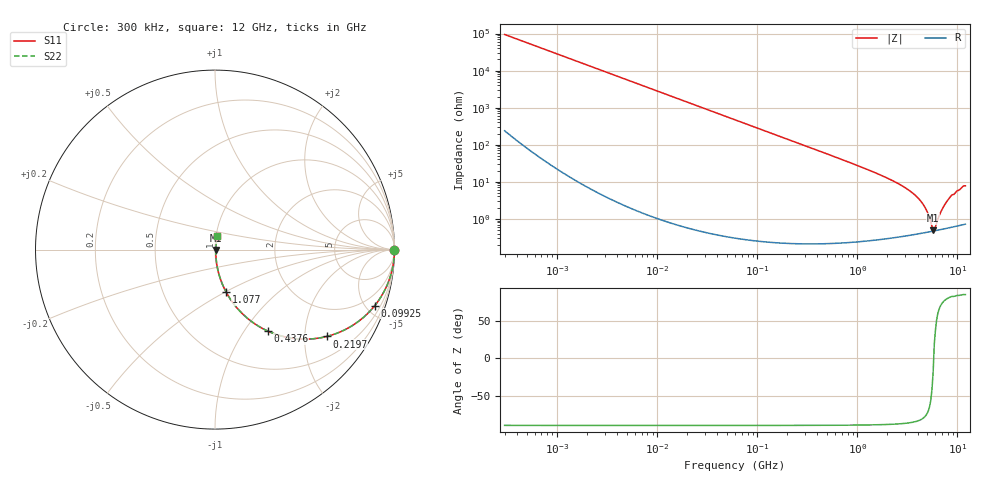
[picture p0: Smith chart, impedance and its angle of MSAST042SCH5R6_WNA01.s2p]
! MSAST042SCH5R6_WNA01  S-PARAMETER MODEL  ( General Type )
! Model Generated by TAIYO YUDEN Corporation (http://www.ty-top.com)
! Version 1.0
! TAIYO YUDEN Control No. 150820
! Copyright(c) 2015 TAIYO YUDEN CO.,LTD. All Rights Reserved.
! Product Description (link to TY-COMPAS)
! https://ds.yuden.co.jp/TYCOMPAS/or/detail?pn=MSAST042SCH5R6BWNA01&u=M
! Products Name : Multilayer Ceramic Capacitors
! Characteristics :
!  Capacitance : 5.6 pF , Rated Voltage : 25V , TCC : CH / C0H
!  Case Size : 0.4 x 0.2 / 0.016 x 0.008 [mm/inch] , Thickness : 0.2 / 0.008 [mm/inch]
!  (Conditions: Temperature = 25 degC , DC Bias Current/Voltage = 0A / 0V)
! External Node Assignments :
!  1  o---| |---o  2
! GND o---------o GND
! Frequency Range : 0.3MHz  -  12000MHz  [ 401 STEP ]
# MHz S RI R 50
! Freq[MHz].  S11 Real  S11 Imag  S21 Real  S21 Imag  S12 Real  S12 Imag  S22 Real  S22 Imag
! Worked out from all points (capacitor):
!   401 points, 300 kHz to 12 GHz, reference 50 ohm
!   read as one part in series: C = 5.62 pF near 316.3 kHz
!   lowest |Z| = 492 mohm at 5.715 GHz (marker M1)
!   series resonance near 5.792 GHz, so ESL is about 130 pH
!   S11 on the Smith chart (normalised r, x): 300 kHz: open; 99.25 MHz: 1.01, -5.71; 219.7 MHz: 1.00, -2.58; 437.6 MHz: 1.00, -1.29; 1.077 GHz: 1.00, -0.51; 12 GHz: 1.01, +0.15
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0.3  1 -0.00106  3.78e-06 0.00106  3.78e-06 0.00106  1 -0.00106
1.769972  1 -0.00625  4.24e-05 0.00625  4.24e-05 0.00625  1 -0.00625
10.44266  0.9986 -0.0368  0.00137 0.0368  0.00137 0.0368  0.9986 -0.0368
27.82928  0.9904 -0.0973  0.00959 0.0973  0.00959 0.0973  0.9904 -0.0973
60  0.957 -0.2026  0.043 0.2026  0.043 0.2026  0.957 -0.2026
99.25425  0.8905 -0.3119  0.1095 0.3119  0.1095 0.3119  0.8905 -0.3119
147.6816  0.7859 -0.4096  0.2141 0.4096  0.2141 0.4096  0.7859 -0.4096
219.7372  0.6236 -0.4836  0.3764 0.4836  0.3764 0.4836  0.6236 -0.4836
353.9943  0.3891 -0.4862  0.6109 0.4862  0.6109 0.4862  0.3891 -0.4862
437.5599  0.2938 -0.4538  0.7062 0.4538  0.7062 0.4538  0.2938 -0.4538
668.5285  0.1502 -0.3547  0.8498 0.3547  0.8498 0.3547  0.1502 -0.3547
1076.992  0.0626 -0.2376  0.9374 0.2376  0.9374 0.2376  0.0626 -0.2376
2088.533  0.0166 -0.1158  0.9834 0.1158  0.9834 0.1158  0.0166 -0.1158
3107.553  0.00763 -0.0643  0.9924 0.0643  0.9924 0.0643  0.00763 -0.0643
4050.141  0.00517 -0.0356  0.9948 0.0356  0.9948 0.0356  0.00517 -0.0356
4747.894  0.0046 -0.0196  0.9954 0.0196  0.9954 0.0196  0.0046 -0.0196
5565.855  0.00459 -0.00406  0.9954 0.00406  0.9954 0.00406  0.00459 -0.00406
5715.274  0.00463 -0.00157  0.9954 0.00157  0.9954 0.00157  0.00463 -0.00157
6026.253  0.00478 0.0036  0.9952 -0.0036  0.9952 -0.0036  0.00478 0.0036
7064.448  0.00551 0.0176  0.9945 -0.0176  0.9945 -0.0176  0.00551 0.0176
8281.503  0.00693 0.0352  0.9931 -0.0352  0.9931 -0.0352  0.00693 0.0352
12000  0.013 0.0759  0.987 -0.0759  0.987 -0.0759  0.013 0.0759
